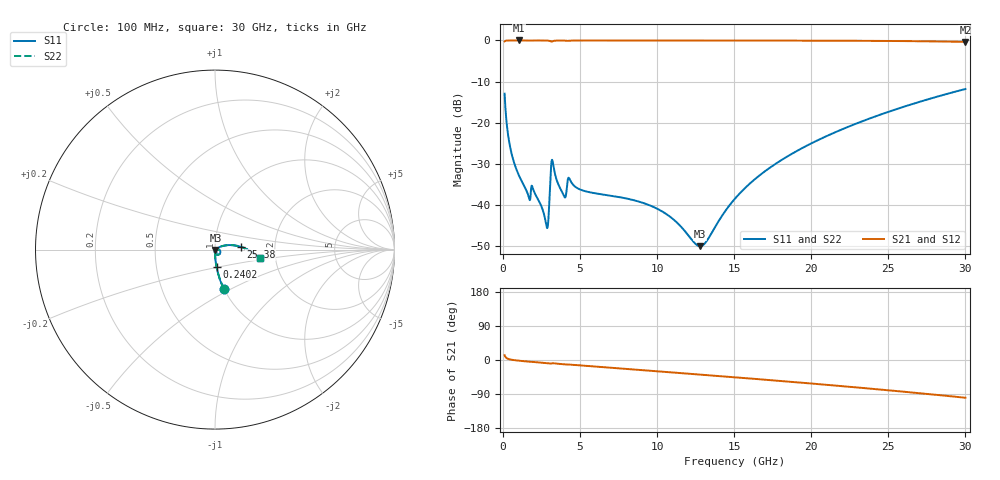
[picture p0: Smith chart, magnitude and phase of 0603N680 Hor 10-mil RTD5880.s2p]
# GHz S MA R 50
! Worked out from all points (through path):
!   3201 points, 100 MHz to 30 GHz, reference 50 ohm
!   highest |S21| = -0.01 dB at 1.034 GHz (marker M1); lowest = -0.4 dB at 30 GHz (marker M2)
!   group delay of S21, straight-line fit = 9.19 ps
!   lowest |S11| = -50.0 dB at 12.79 GHz (marker M3), VSWR 1.01, Z = 50.2 - j0.205 ohm
!   |S11| at or under -10 dB: start of sweep to end of sweep
!   |S22| runs from -50.0 to -11.8 dB; largest |S21 - S12| = 0
!   S11 on the Smith chart (normalised r, x): 100 MHz: 1.00, -0.46; 240.2 MHz: 1.00, -0.19; 25.38 GHz: 1.33, +0.04; 30 GHz: 1.66, -0.18
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0.1  0.225 -77.2  0.974 12.7  0.974 12.7  0.225 -77.2
0.2401562  0.09583 -85.0  0.995 4.8  0.995 4.8  0.09583 -85.0
0.5298125  0.04384 -88.3  0.9984 0.9  0.9984 0.9  0.04384 -88.3
1.034375  0.02275 -89.7  0.9989 -1.9  0.9989 -1.9  0.02275 -89.7
1.641719  0.01295 -86.3  0.9981 -4.3  0.9981 -4.3  0.01295 -86.3
1.978094  0.01506 -85.8  0.9974 -5.2  0.9974 -5.2  0.01506 -85.8
2.800344  0.005753 -62.4  0.9966 -8.3  0.9966 -8.3  0.005753 -62.4
2.912469  0.00572 -21.5  0.9944 -8.9  0.9944 -8.9  0.00572 -21.5
3.118031  0.02962 -14.0  0.9704 -9.4  0.9704 -9.4  0.02962 -14.0
3.230156  0.03283 -60.8  0.9796 -8.4  0.9796 -8.4  0.03283 -60.8
3.930938  0.01304 -83.3  0.9958 -11.3  0.9958 -11.3  0.01304 -83.3
4.314031  0.02073 -83.6  0.9932 -12.1  0.9932 -12.1  0.02073 -83.6
5.089563  0.01518 -96.0  0.9975 -14.7  0.9975 -14.7  0.01518 -96.0
10.06978  0.008863 -102.0  0.9971 -30.1  0.9971 -30.1  0.008863 -102.0
12.78881  0.003155 -40.4  0.9967 -38.5  0.9967 -38.5  0.003155 -40.4
13.19994  0.003615 -12.7  0.9966 -39.8  0.9966 -39.8  0.003615 -12.7
15.05  0.01194 27.2  0.9962 -45.7  0.9962 -45.7  0.01194 27.2
17.143  0.02691 29.2  0.9955 -52.5  0.9955 -52.5  0.02691 29.2
20.03956  0.05649 23.3  0.9937 -62.2  0.9937 -62.2  0.05649 23.3
25.01978  0.1358 7.7  0.9849 -80.0  0.9849 -80.0  0.1358 7.7
25.38419  0.1431 6.4  0.9838 -81.3  0.9838 -81.3  0.1431 6.4
30  0.2567 -11.1  0.9594 -99.6  0.9594 -99.6  0.2567 -11.1
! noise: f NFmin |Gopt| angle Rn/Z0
0.1  0.0002865  0.9169  0.3572  0.0007606
3.417  0.006619  0.8797  10.49  0.01181
6.743  0.005816  0.7503  20.63  0.004547
10.06  0.007746  0.7271  30.55  0.005262
13.39  0.009666  0.7151  40.25  0.005929
16.7  0.01159  0.7095  49.64  0.006509
20.03  0.01357  0.7083  58.73  0.007016
23.35  0.01565  0.7105  67.45  0.007457
26.67  0.01787  0.7154  75.85  0.007844
30  0.02028  0.7224  83.91  0.00818
